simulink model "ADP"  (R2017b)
settings: Solver=FixedStepDiscrete  StartTime=0.0  StopTime=10.0  FixedStep=0.01  RelTol=1e-3  EnableMultiTasking=on
undefined symbols (not defined in the file): ADP050_RUNTIME_MS, ADP195_RUNTIME_MS, ADP_CONST100_NUMB, ADP_CONST2147483648_NUMB, ADP_CONST3_NUMB, ADP_CONST80_NUMB, ASWTYPE_FALSE, ASWTYPE_TRUE, CcADP_ABMDiagKL15DelayTi_ms, CcADP_ObcCmdto0Ti_ms, Enum_ADPStopChgReq, Enum_ISPDischgReq, Enum_LDPCC2St, Enum_MSMBMUState, Enum_ODPCCState, Enum_UDSPrjSel
libraries: AIWAYS_Powertrain_BMS_lib x68
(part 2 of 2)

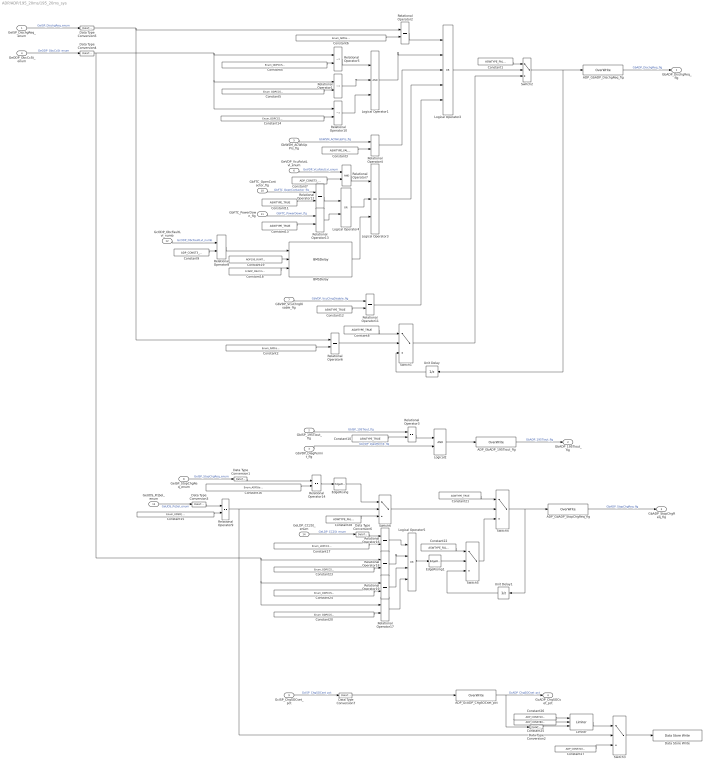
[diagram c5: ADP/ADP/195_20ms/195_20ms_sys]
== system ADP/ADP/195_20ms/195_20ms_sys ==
  GeISP_DischgReq_enum : Inport
  GbISP_195Tiout_flg : Inport  Port=2
  GbVDP_DiagPermit_flg : Inport  Port=3
  GeODP_ObcCcSt_enum : Inport  Port=4
  GbWSM_ACWkUpPrs_flg : Inport  Port=5
  GeVDP_VcuFalutLvl_enum : Inport  Port=6
  GbVDP_VcuChrgDisable_flg : Inport  Port=7
  GeISP_StopChgReq_enum : Inport  Port=8
  GcISP_ChgSOCset_pct : Inport  Port=9
  GbFTC_OpenContactor_flg : Inport  Port=10
  GbFTC_PowerDown_flg : Inport  Port=11
  GcODP_ObcFaultLvl_numb : Inport  Port=12
  GeUDS_PrjSel_enum : Inport  Port=13
  GeLDP_CC2St_enum : Inport  Port=14
  ADP_GbADP_195Tiout_flg : AIWAYS_Powertrain_BMS_lib/Signals/OverWrite  OverWrite_Value=CbADP_195TioutOvr_flg  OverWrite_flag=CbADP_195TioutOvrSwt_flg
  ADP_GbADP_DischgReq_flg : AIWAYS_Powertrain_BMS_lib/Signals/OverWrite  OverWrite_Value=CbADP_DischgReqOvr_flg  OverWrite_flag=CbADP_DischgReqOvrSwt_flg
  ADP_GbADP_StopChgReq_flg : AIWAYS_Powertrain_BMS_lib/Signals/OverWrite  OverWrite_Value=CbADP_StopChgReqOvr_flg  OverWrite_flag=CbADP_StopChgReqOvrSwt_flg
  ADP_GcADP_ChgSOCset_pct : AIWAYS_Powertrain_BMS_lib/Signals/OverWrite  OverWrite_Value=CcADP_ChgSOCsetOvr_pct  OverWrite_flag=CbADP_ChgSOCsetOvrSwt_flg
  BMSDelay : AIWAYS_Powertrain_BMS_lib/Debounce & Delay/BMSDelay
  Constant{1,3,22,28} (4 alike) : Constant  Value=ASWTYPE_FALSE
  Constant{8,10..13,21} (6 alike) : Constant  Value=ASWTYPE_TRUE
  Constant14 : Constant  Value=Enum_ODPCCState.Enum_ODPCCState_DisChrgConnect32A1000
  Constant15 : Constant  Value=Enum_UDSPrjSel.Enum_UDSPrjSel_891
  Constant16 : Constant  Value=Enum_ADPStopChgReq.Enum_ADPStopChgReq_StopChgReq
  Constant17 : Constant  Value=Enum_LDPCC2St.Enum_LDPCC2St_Connect
  Constant18 : Constant  Value=CcADP_ObcCmdto0Ti_ms
  Constant19 : Constant  Value=ADP195_RUNTIME_MS
  Constant2 : Constant  Value=Enum_ISPDischgReq.Enum_ISPDischgReq_V2XDischrg
  Constant20 : Constant  Value=Enum_ODPCCState.Enum_ODPCCState_ChrgConnect32A220
  Constant23 : Constant  Value=Enum_ODPCCState.Enum_ODPCCState_ChrgConnect10A1500
  Constant24 : Constant  Value=Enum_ODPCCState.Enum_ODPCCState_ChrgConnect16A680
  Constant25 : Constant  Value=ADP_CONST80_NUMB
  Constant26 : Constant  Value=ADP_CONST100_NUMB
  Constant27 : Constant  Value=ADP_CONST100_NUMB
  Constant4 : Constant  Value=Enum_ODPCCState.Enum_ODPCCState_DisChrgConnect10A2700
  Constant5 : Constant  Value=Enum_ODPCCState.Enum_ODPCCState_DisChrgConnect16A2000
  Constant6 : Constant  Value=Enum_ISPDischgReq.Enum_ISPDischgReq_QuitRequest
  Constant7 : Constant  Value=ADP_CONST3_NUMB
  Constant9 : Constant  Value=ADP_CONST3_NUMB
  Data Store Write : AIWAYS_Powertrain_BMS_lib/Signals/Data Store Write  DSW=EcNVM_ChrgPermitMaxSOC_pct
  Data Type Conversion{1..7} (7 alike) : DataTypeConversion
  EdgeRising : AIWAYS_Powertrain_BMS_lib/Logical Operators/EdgeRising
  EdgeRising1 : AIWAYS_Powertrain_BMS_lib/Logical Operators/EdgeRising
  Limiter : AIWAYS_Powertrain_BMS_lib/Nonlinear Blocks/Limiter
  Logical Operator1 : Logic  Inputs=3  AllPortsSameDT=off  OutDataTypeStr=boolean
  Logical Operator2 : Logic  Operator=OR  Inputs=5  AllPortsSameDT=off  OutDataTypeStr=boolean
  Logical Operator3 : Logic  Operator=OR  Inputs=3  AllPortsSameDT=off  OutDataTypeStr=boolean
  Logical Operator4 : Logic  Operator=OR  AllPortsSameDT=off  OutDataTypeStr=boolean
  Logical Operator5 : Logic  Operator=OR  Inputs=4  AllPortsSameDT=off  OutDataTypeStr=boolean
  Logical2 : Logic  OutDataTypeStr=boolean
  Relational Operator1 : RelationalOperator  Operator=~=  OutDataTypeStr=boolean
  Relational Operator10 : RelationalOperator  Operator=~=  OutDataTypeStr=boolean
  Relational Operator{2..4,6,8..9,11..14,16..19} (14 alike) : RelationalOperator  Operator===  OutDataTypeStr=boolean
  Relational Operator5 : RelationalOperator  Operator=~=  OutDataTypeStr=boolean
  Relational Operator7 : RelationalOperator  OutDataTypeStr=boolean
  Switch{1..6} (6 alike) : Switch  Criteria=u2 ~= 0
  Unit Delay : UnitDelay  SampleTime=-1  StateName=StateName
  Unit Delay1 : UnitDelay  SampleTime=-1  StateName=StateName
  GbADP_DischgReq_flg : Outport
  GbADP_195Tiout_flg : Outport  Port=2
  GbADP_StopChgReq_flg : Outport  Port=3
  GcADP_ChgSOCset_pct : Outport  Port=4
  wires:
  GbISP_195Tiout_flg/1 -> Relational Operator3/1  "GbISP_195Tiout_flg"
  GeISP_DischgReq_enum/1 -> Data Type Conversion5/1  "GeISP_DischgReq_enum"
  ADP_GbADP_DischgReq_flg/1 -> GbADP_DischgReq_flg/1  "GbADP_DischgReq_flg"
  GbVDP_DiagPermit_flg/1 -> Logical2/2  "GbVDP_DiagPermit_flg"
  Logical2/1 -> ADP_GbADP_195Tiout_flg/1
  Constant10/1 -> Relational Operator3/2
  Relational Operator3/1 -> Logical2/1
  ADP_GbADP_195Tiout_flg/1 -> GbADP_195Tiout_flg/1  "GbADP_195Tiout_flg"
  Relational Operator6/1 -> Switch1/2
  Constant2/1 -> Relational Operator6/2
  Constant8/1 -> Switch1/1
  Switch1/1 -> Switch2/3
  Constant1/1 -> Switch2/1
  Switch2/1 -> ADP_GbADP_DischgReq_flg/1, Unit Delay/1
  Unit Delay/1 -> Switch1/3
  Logical Operator2/1 -> Switch2/2
  Relational Operator5/1 -> Logical Operator1/1
  Constant4/1 -> Relational Operator5/2
  Constant14/1 -> Relational Operator10/2
  Relational Operator1/1 -> Logical Operator1/2
  Relational Operator10/1 -> Logical Operator1/3
  Constant5/1 -> Relational Operator1/2
  GeODP_ObcCcSt_enum/1 -> Data Type Conversion4/1  "GeODP_ObcCcSt_enum"
  Constant6/1 -> Relational Operator2/2
  GbWSM_ACWkUpPrs_flg/1 -> Relational Operator4/1  "GbWSM_ACWkUpPrs_flg"
  Constant3/1 -> Relational Operator4/2
  Relational Operator2/1 -> Logical Operator2/1
  Logical Operator1/1 -> Logical Operator2/2
  Relational Operator4/1 -> Logical Operator2/3
  GeVDP_VcuFalutLvl_enum/1 -> Relational Operator7/1  "GeVDP_VcuFalutLvl_enum"
  Constant7/1 -> Relational Operator7/2
  Relational Operator7/1 -> Logical Operator3/1
  Logical Operator4/1 -> Logical Operator3/2
  Logical Operator3/1 -> Logical Operator2/4
  GbVDP_VcuChrgDisable_flg/1 -> Relational Operator11/1  "GbVDP_VcuChrgDisable_flg"
  Constant12/1 -> Relational Operator11/2
  Relational Operator11/1 -> Logical Operator2/5
  Data Type Conversion5/1 -> Relational Operator6/1, Relational Operator2/1
  GeISP_StopChgReq_enum/1 -> Data Type Conversion1/1  "GeISP_StopChgReq_enum"
  GcISP_ChgSOCset_pct/1 -> Data Type Conversion7/1  "GcISP_ChgSOCset_pct"
  Data Type Conversion1/1 -> Relational Operator14/1
  ADP_GbADP_StopChgReq_flg/1 -> GbADP_StopChgReq_flg/1  "GbADP_StopChgReq_flg"
  Data Type Conversion7/1 -> ADP_GcADP_ChgSOCset_pct/1
  ADP_GcADP_ChgSOCset_pct/1 -> GcADP_ChgSOCset_pct/1, Data Type Conversion2/1  "GcADP_ChgSOCset_pct"
  GbFTC_OpenContactor_flg/1 -> Relational Operator12/1  "GbFTC_OpenContactor_flg"
  Relational Operator13/1 -> Logical Operator4/2
  Constant13/1 -> Relational Operator13/2
  Constant11/1 -> Relational Operator12/2
  GbFTC_PowerDown_flg/1 -> Relational Operator13/1  "GbFTC_PowerDown_flg"
  Relational Operator12/1 -> Logical Operator4/1
  GcODP_ObcFaultLvl_numb/1 -> Relational Operator8/1  "GcODP_ObcFaultLvl_numb"
  Relational Operator8/1 -> BMSDelay/1
  Constant9/1 -> Relational Operator8/2
  Constant19/1 -> BMSDelay/2
  Constant18/1 -> BMSDelay/3
  BMSDelay/1 -> Logical Operator3/3
  Data Type Conversion2/1 -> Limiter/3
  Constant15/1 -> Relational Operator9/2
  Data Type Conversion3/1 -> Relational Operator9/1
  GeUDS_PrjSel_enum/1 -> Data Type Conversion3/1  "GeUDS_PrjSel_enum"
  Relational Operator9/1 -> Switch3/2, Switch6/2
  Switch3/1 -> Data Store Write/1
  Constant27/1 -> Switch3/3
  Constant16/1 -> Relational Operator14/2
  Relational Operator14/1 -> EdgeRising/1
  Constant21/1 -> Switch4/1
  EdgeRising/1 -> Switch6/1
  Unit Delay1/1 -> Switch5/3
  Constant17/1 -> Relational Operator16/2
  EdgeRising1/1 -> Switch5/2
  Switch4/1 -> ADP_GbADP_StopChgReq_flg/1, Unit Delay1/1
  Relational Operator16/1 -> Logical Operator5/1
  Switch5/1 -> Switch4/3
  Constant22/1 -> Switch5/1
  Data Type Conversion6/1 -> Relational Operator16/1
  GeLDP_CC2St_enum/1 -> Data Type Conversion6/1  "GeLDP_CC2St_enum"
  Logical Operator5/1 -> EdgeRising1/1
  Relational Operator18/1 -> Logical Operator5/2
  Constant20/1 -> Relational Operator17/2
  Constant24/1 -> Relational Operator19/2
  Data Type Conversion4/1 -> Relational Operator18/1, Relational Operator17/1, Relational Operator19/1, Relational Operator5/1, Relational Operator10/1, Relational Operator1/1
  Constant23/1 -> Relational Operator18/2
  Relational Operator19/1 -> Logical Operator5/3
  Relational Operator17/1 -> Logical Operator5/4
  Limiter/1 -> Switch3/1
  Constant25/1 -> Limiter/2
  Constant26/1 -> Limiter/1
  Switch6/1 -> Switch4/2
  Constant28/1 -> Switch6/3

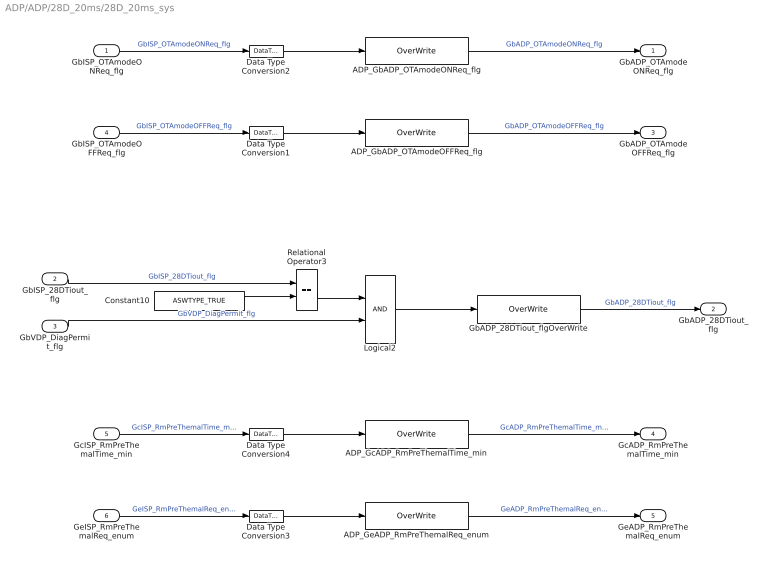
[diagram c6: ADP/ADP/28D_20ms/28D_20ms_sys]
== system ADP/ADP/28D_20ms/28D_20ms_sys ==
  GbISP_OTAmodeONReq_flg : Inport
  GbISP_28DTiout_flg : Inport  Port=2
  GbVDP_DiagPermit_flg : Inport  Port=3
  GbISP_OTAmodeOFFReq_flg : Inport  Port=4
  GcISP_RmPreThemalTime_min : Inport  Port=5
  GeISP_RmPreThemalReq_enum : Inport  Port=6
  ADP_GbADP_OTAmodeOFFReq_flg : AIWAYS_Powertrain_BMS_lib/Signals/OverWrite  OverWrite_Value=CbADP_OTAmodeOFFReqOvr_flg  OverWrite_flag=CbADP_OTAmodeOFFReqOvrSwt_flg
  ADP_GbADP_OTAmodeONReq_flg : AIWAYS_Powertrain_BMS_lib/Signals/OverWrite  OverWrite_Value=CbADP_OTAmodeONReqOvr_flg  OverWrite_flag=CbADP_OTAmodeONReqOvrSwt_flg
  ADP_GcADP_RmPreThemalTime_min : AIWAYS_Powertrain_BMS_lib/Signals/OverWrite  OverWrite_Value=CcADP_RmPreThemalTimeOvr_min  OverWrite_flag=CbADP_RmPreThemalTimeOvrSwt_flg
  ADP_GeADP_RmPreThemalReq_enum : AIWAYS_Powertrain_BMS_lib/Signals/OverWrite  OverWrite_Value=CeADP_RmPreThemalReqOvr_enum  OverWrite_flag=CbADP_RmPreThemalReqOvrSwt_flg
  Constant10 : Constant  Value=ASWTYPE_TRUE
  Data Type Conversion{1..4} (4 alike) : DataTypeConversion
  GbADP_28DTiout_flgOverWrite : AIWAYS_Powertrain_BMS_lib/Signals/OverWrite  OverWrite_Value=CbADP_28DTioutOvr_flg  OverWrite_flag=CbADP_28DTioutOvrSwt_flg
  Logical2 : Logic  OutDataTypeStr=boolean
  Relational Operator3 : RelationalOperator  Operator===  OutDataTypeStr=boolean
  GbADP_OTAmodeONReq_flg : Outport
  GbADP_28DTiout_flg : Outport  Port=2
  GbADP_OTAmodeOFFReq_flg : Outport  Port=3
  GcADP_RmPreThemalTime_min : Outport  Port=4
  GeADP_RmPreThemalReq_enum : Outport  Port=5
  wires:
  GbISP_OTAmodeONReq_flg/1 -> Data Type Conversion2/1  "GbISP_OTAmodeONReq_flg"
  GbISP_28DTiout_flg/1 -> Relational Operator3/1  "GbISP_28DTiout_flg"
  ADP_GbADP_OTAmodeONReq_flg/1 -> GbADP_OTAmodeONReq_flg/1  "GbADP_OTAmodeONReq_flg"
  GbVDP_DiagPermit_flg/1 -> Logical2/2  "GbVDP_DiagPermit_flg"
  Constant10/1 -> Relational Operator3/2
  Logical2/1 -> GbADP_28DTiout_flgOverWrite/1
  Relational Operator3/1 -> Logical2/1
  ADP_GbADP_OTAmodeOFFReq_flg/1 -> GbADP_OTAmodeOFFReq_flg/1  "GbADP_OTAmodeOFFReq_flg"
  GbISP_OTAmodeOFFReq_flg/1 -> Data Type Conversion1/1  "GbISP_OTAmodeOFFReq_flg"
  GbADP_28DTiout_flgOverWrite/1 -> GbADP_28DTiout_flg/1  "GbADP_28DTiout_flg"
  Data Type Conversion2/1 -> ADP_GbADP_OTAmodeONReq_flg/1
  Data Type Conversion1/1 -> ADP_GbADP_OTAmodeOFFReq_flg/1
  GeISP_RmPreThemalReq_enum/1 -> Data Type Conversion3/1  "GeISP_RmPreThemalReq_enum"
  Data Type Conversion4/1 -> ADP_GcADP_RmPreThemalTime_min/1
  Data Type Conversion3/1 -> ADP_GeADP_RmPreThemalReq_enum/1
  GcISP_RmPreThemalTime_min/1 -> Data Type Conversion4/1  "GcISP_RmPreThemalTime_min"
  ADP_GcADP_RmPreThemalTime_min/1 -> GcADP_RmPreThemalTime_min/1  "GcADP_RmPreThemalTime_min"
  ADP_GeADP_RmPreThemalReq_enum/1 -> GeADP_RmPreThemalReq_enum/1  "GeADP_RmPreThemalReq_enum"

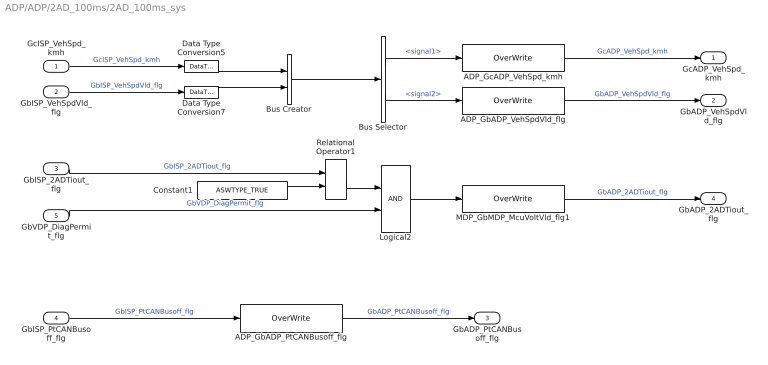
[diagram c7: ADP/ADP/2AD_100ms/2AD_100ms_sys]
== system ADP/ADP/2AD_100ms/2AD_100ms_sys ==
  GcISP_VehSpd_kmh : Inport
  GbISP_VehSpdVld_flg : Inport  Port=2
  GbISP_2ADTiout_flg : Inport  Port=3
  GbISP_PtCANBusoff_flg : Inport  Port=4
  GbVDP_DiagPermit_flg : Inport  Port=5
  ADP_GbADP_PtCANBusoff_flg : AIWAYS_Powertrain_BMS_lib/Signals/OverWrite  OverWrite_Value=CbADP_PtCANBusoffOvr_flg  OverWrite_flag=CbADP_PtCANBusoffOvrSwt_flg
  ADP_GbADP_VehSpdVld_flg : AIWAYS_Powertrain_BMS_lib/Signals/OverWrite  OverWrite_Value=CbADP_VehSpdVldOvr_flg  OverWrite_flag=CbADP_VehSpdVldOvrSwt_flg
  ADP_GcADP_VehSpd_kmh : AIWAYS_Powertrain_BMS_lib/Signals/OverWrite  OverWrite_Value=CcADP_VehSpdOvr_kmh  OverWrite_flag=CbADP_VehSpdOvrSwt_flg
  Bus Creator : BusCreator  Inputs=2
  Bus Selector : BusSelector  OutputSignals=signal1,signal2
  Constant1 : Constant  Value=ASWTYPE_TRUE
  Data Type Conversion5 : DataTypeConversion
  Data Type Conversion7 : DataTypeConversion
  Logical2 : Logic  OutDataTypeStr=boolean
  MDP_GbMDP_McuVoltVld_flg1 : AIWAYS_Powertrain_BMS_lib/Signals/OverWrite  OverWrite_Value=CbADP_2ADTioutOvr_flg  OverWrite_flag=CbADP_2ADTioutOvrSwt_flg
  Relational Operator1 : RelationalOperator  Operator===  OutDataTypeStr=boolean
  GcADP_VehSpd_kmh : Outport
  GbADP_VehSpdVld_flg : Outport  Port=2
  GbADP_PtCANBusoff_flg : Outport  Port=3
  GbADP_2ADTiout_flg : Outport  Port=4
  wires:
  Bus Selector/2 -> ADP_GbADP_VehSpdVld_flg/1  "<signal2>"
  Data Type Conversion5/1 -> Bus Creator/1
  Data Type Conversion7/1 -> Bus Creator/2
  Bus Creator/1 -> Bus Selector/1
  Bus Selector/1 -> ADP_GcADP_VehSpd_kmh/1  "<signal1>"
  GcISP_VehSpd_kmh/1 -> Data Type Conversion5/1  "GcISP_VehSpd_kmh"
  GbISP_VehSpdVld_flg/1 -> Data Type Conversion7/1  "GbISP_VehSpdVld_flg"
  GbISP_2ADTiout_flg/1 -> Relational Operator1/1  "GbISP_2ADTiout_flg"
  ADP_GcADP_VehSpd_kmh/1 -> GcADP_VehSpd_kmh/1  "GcADP_VehSpd_kmh"
  ADP_GbADP_VehSpdVld_flg/1 -> GbADP_VehSpdVld_flg/1  "GbADP_VehSpdVld_flg"
  ADP_GbADP_PtCANBusoff_flg/1 -> GbADP_PtCANBusoff_flg/1  "GbADP_PtCANBusoff_flg"
  GbISP_PtCANBusoff_flg/1 -> ADP_GbADP_PtCANBusoff_flg/1  "GbISP_PtCANBusoff_flg"
  Logical2/1 -> MDP_GbMDP_McuVoltVld_flg1/1
  GbVDP_DiagPermit_flg/1 -> Logical2/2  "GbVDP_DiagPermit_flg"
  MDP_GbMDP_McuVoltVld_flg1/1 -> GbADP_2ADTiout_flg/1  "GbADP_2ADTiout_flg"
  Constant1/1 -> Relational Operator1/2
  Relational Operator1/1 -> Logical2/1

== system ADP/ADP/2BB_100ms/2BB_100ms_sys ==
  GcISP_EnvT_C : Inport
  GbISP_2BBTiout_flg : Inport  Port=2
  GbVDP_DiagPermit_flg : Inport  Port=3
  ADP_GbADP_2BBTiout_flg : AIWAYS_Powertrain_BMS_lib/Signals/OverWrite  OverWrite_Value=CbADP_2BBTioutOvr_flg  OverWrite_flag=CbADP_2BBTioutOvrSwt_flg
  ADP_GcADP_EnvT_C : AIWAYS_Powertrain_BMS_lib/Signals/OverWrite  OverWrite_Value=CcADP_EnvTOvr_C  OverWrite_flag=CbADP_EnvTOvrSwt_flg
  Constant1 : Constant  Value=ASWTYPE_TRUE
  Data Type Conversion5 : DataTypeConversion
  Logical2 : Logic  OutDataTypeStr=boolean
  Relational Operator1 : RelationalOperator  Operator===  OutDataTypeStr=boolean
  GcADP_EnvT_C : Outport
  GbADP_2BBTiout_flg : Outport  Port=2
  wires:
  GbISP_2BBTiout_flg/1 -> Relational Operator1/1  "GbISP_2BBTiout_flg"
  GcISP_EnvT_C/1 -> Data Type Conversion5/1  "GcISP_EnvT_C"
  Data Type Conversion5/1 -> ADP_GcADP_EnvT_C/1
  ADP_GcADP_EnvT_C/1 -> GcADP_EnvT_C/1  "GcADP_EnvT_C"
  Logical2/1 -> ADP_GbADP_2BBTiout_flg/1
  GbVDP_DiagPermit_flg/1 -> Logical2/2  "GbVDP_DiagPermit_flg"
  Constant1/1 -> Relational Operator1/2
  Relational Operator1/1 -> Logical2/1
  ADP_GbADP_2BBTiout_flg/1 -> GbADP_2BBTiout_flg/1  "GbADP_2BBTiout_flg"

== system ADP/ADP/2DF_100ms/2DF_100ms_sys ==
  GcISP_AcmDist_numb : Inport
  GbISP_AcmDistVld_flg : Inport  Port=2
  GbISP_2DFTiout_flg : Inport  Port=3
  GbVDP_DiagPermit_flg : Inport  Port=4
  ADP_GbADP_2DFTiout_flg : AIWAYS_Powertrain_BMS_lib/Signals/OverWrite  OverWrite_Value=CbADP_2DFTioutOvr_flg  OverWrite_flag=CbADP_2DFTioutOvrSwt_flg
  ADP_GbADP_AcmDistVld_flg : AIWAYS_Powertrain_BMS_lib/Signals/OverWrite  OverWrite_Value=CbADP_AcmDistVldOvr_flg  OverWrite_flag=CbADP_AcmDistVldOvrSwt_flg
  ADP_GcADP_AcmDist_numb : AIWAYS_Powertrain_BMS_lib/Signals/OverWrite  OverWrite_Value=CcADP_AcmDistOvr_numb  OverWrite_flag=CbADP_AcmDistOvrSwt_flg
  Bus Creator : BusCreator  Inputs=2
  Bus Selector : BusSelector  OutputSignals=signal1,signal2
  Constant3 : Constant  Value=ASWTYPE_TRUE
  Data Type Conversion5 : DataTypeConversion
  Data Type Conversion7 : DataTypeConversion
  Logical2 : Logic  OutDataTypeStr=boolean
  Relational Operator1 : RelationalOperator  Operator===  OutDataTypeStr=boolean
  GcADP_AcmDist_numb : Outport
  GbADP_AcmDistVld_flg : Outport  Port=2
  GbADP_2DFTiout_flg : Outport  Port=3
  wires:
  Bus Selector/1 -> ADP_GcADP_AcmDist_numb/1  "<signal1>"
  Bus Selector/2 -> ADP_GbADP_AcmDistVld_flg/1  "<signal2>"
  Bus Creator/1 -> Bus Selector/1
  Data Type Conversion7/1 -> Bus Creator/2
  Data Type Conversion5/1 -> Bus Creator/1
  GcISP_AcmDist_numb/1 -> Data Type Conversion5/1  "GcISP_AcmDist_numb"
  GbISP_AcmDistVld_flg/1 -> Data Type Conversion7/1  "GbISP_AcmDistVld_flg"
  GbISP_2DFTiout_flg/1 -> Relational Operator1/1  "GbISP_2DFTiout_flg"
  ADP_GcADP_AcmDist_numb/1 -> GcADP_AcmDist_numb/1  "GcADP_AcmDist_numb"
  ADP_GbADP_AcmDistVld_flg/1 -> GbADP_AcmDistVld_flg/1  "GbADP_AcmDistVld_flg"
  GbVDP_DiagPermit_flg/1 -> Logical2/2  "GbVDP_DiagPermit_flg"
  Logical2/1 -> ADP_GbADP_2DFTiout_flg/1
  Constant3/1 -> Relational Operator1/2
  Relational Operator1/1 -> Logical2/1
  ADP_GbADP_2DFTiout_flg/1 -> GbADP_2DFTiout_flg/1  "GbADP_2DFTiout_flg"

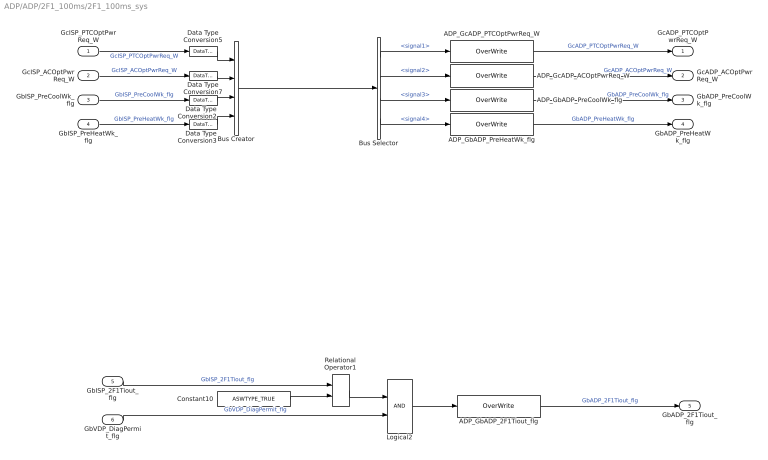
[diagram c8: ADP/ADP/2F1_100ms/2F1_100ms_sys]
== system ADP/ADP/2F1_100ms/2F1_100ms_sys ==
  GcISP_PTCOptPwrReq_W : Inport
  GcISP_ACOptPwrReq_W : Inport  Port=2
  GbISP_PreCoolWk_flg : Inport  Port=3
  GbISP_PreHeatWk_flg : Inport  Port=4
  GbISP_2F1Tiout_flg : Inport  Port=5
  GbVDP_DiagPermit_flg : Inport  Port=6
  ADP_GbADP_2F1Tiout_flg : AIWAYS_Powertrain_BMS_lib/Signals/OverWrite  OverWrite_Value=CbADP_2F1TioutOvr_flg  OverWrite_flag=CbADP_2F1TioutOvrSwt_flg
  ADP_GbADP_PreCoolWk_flg : AIWAYS_Powertrain_BMS_lib/Signals/OverWrite  OverWrite_Value=CbADP_PreCoolWkOvr_flg  OverWrite_flag=CbADP_PreCoolWkOvrSwt_flg
  ADP_GbADP_PreHeatWk_flg : AIWAYS_Powertrain_BMS_lib/Signals/OverWrite  OverWrite_Value=CbADP_PreHeatWkOvr_flg  OverWrite_flag=CbADP_PreHeatWkOvrSwt_flg
  ADP_GcADP_ACOptPwrReq_W : AIWAYS_Powertrain_BMS_lib/Signals/OverWrite  OverWrite_Value=CcADP_ACOptPwrReqOvr_W  OverWrite_flag=CbADP_ACOptPwrReqOvrSwt_flg
  ADP_GcADP_PTCOptPwrReq_W : AIWAYS_Powertrain_BMS_lib/Signals/OverWrite  OverWrite_Value=CcADP_PTCOptPwrReqOvr_W  OverWrite_flag=CbADP_PTCOptPwrReqOvrSwt_flg
  Bus Creator : BusCreator  Inputs=4
  Bus Selector : BusSelector  OutputSignals=signal1,signal2,signal3,signal4
  Constant10 : Constant  Value=ASWTYPE_TRUE
  Data Type Conversion{2..3,5,7} (4 alike) : DataTypeConversion
  Logical2 : Logic  OutDataTypeStr=boolean
  Relational Operator1 : RelationalOperator  Operator===  OutDataTypeStr=boolean
  GcADP_PTCOptPwrReq_W : Outport
  GcADP_ACOptPwrReq_W : Outport  Port=2
  GbADP_PreCoolWk_flg : Outport  Port=3
  GbADP_PreHeatWk_flg : Outport  Port=4
  GbADP_2F1Tiout_flg : Outport  Port=5
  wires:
  Bus Creator/1 -> Bus Selector/1
  Data Type Conversion7/1 -> Bus Creator/2
  Data Type Conversion5/1 -> Bus Creator/1
  GcISP_ACOptPwrReq_W/1 -> Data Type Conversion7/1  "GcISP_ACOptPwrReq_W"
  GcISP_PTCOptPwrReq_W/1 -> Data Type Conversion5/1  "GcISP_PTCOptPwrReq_W"
  GbISP_PreCoolWk_flg/1 -> Data Type Conversion2/1  "GbISP_PreCoolWk_flg"
  GbISP_PreHeatWk_flg/1 -> Data Type Conversion3/1  "GbISP_PreHeatWk_flg"
  GbISP_2F1Tiout_flg/1 -> Relational Operator1/1  "GbISP_2F1Tiout_flg"
  ADP_GcADP_PTCOptPwrReq_W/1 -> GcADP_PTCOptPwrReq_W/1  "GcADP_PTCOptPwrReq_W"
  ADP_GcADP_ACOptPwrReq_W/1 -> GcADP_ACOptPwrReq_W/1  "GcADP_ACOptPwrReq_W"
  ADP_GbADP_PreCoolWk_flg/1 -> GbADP_PreCoolWk_flg/1  "GbADP_PreCoolWk_flg"
  ADP_GbADP_PreHeatWk_flg/1 -> GbADP_PreHeatWk_flg/1  "GbADP_PreHeatWk_flg"
  Bus Selector/1 -> ADP_GcADP_PTCOptPwrReq_W/1  "<signal1>"
  Bus Selector/2 -> ADP_GcADP_ACOptPwrReq_W/1  "<signal2>"
  Bus Selector/3 -> ADP_GbADP_PreCoolWk_flg/1  "<signal3>"
  Bus Selector/4 -> ADP_GbADP_PreHeatWk_flg/1  "<signal4>"
  Data Type Conversion2/1 -> Bus Creator/3
  Data Type Conversion3/1 -> Bus Creator/4
  Logical2/1 -> ADP_GbADP_2F1Tiout_flg/1
  GbVDP_DiagPermit_flg/1 -> Logical2/2  "GbVDP_DiagPermit_flg"
  Relational Operator1/1 -> Logical2/1
  Constant10/1 -> Relational Operator1/2
  ADP_GbADP_2F1Tiout_flg/1 -> GbADP_2F1Tiout_flg/1  "GbADP_2F1Tiout_flg"

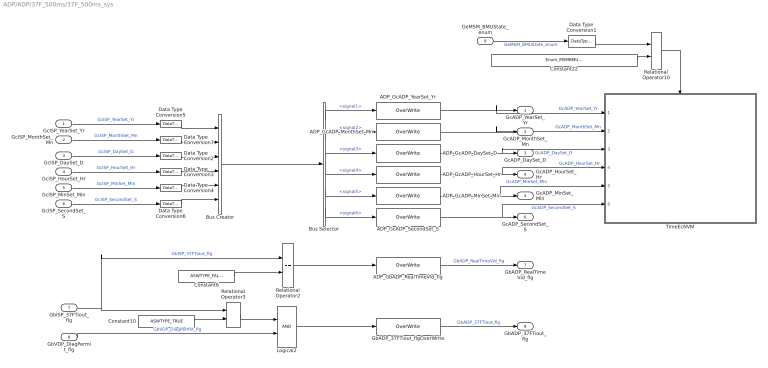
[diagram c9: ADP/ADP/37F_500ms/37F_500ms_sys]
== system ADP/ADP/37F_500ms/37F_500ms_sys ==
  GcISP_YearSet_Yr : Inport
  GcISP_MonthSet_Mn : Inport  Port=2
  GcISP_DaySet_D : Inport  Port=3
  GcISP_HourSet_Hr : Inport  Port=4
  GcISP_MinSet_Min : Inport  Port=5
  GcISP_SecondSet_S : Inport  Port=6
  GbISP_37FTiout_flg : Inport  Port=7
  GbVDP_DiagPermit_flg : Inport  Port=8
  GeMSM_BMUState_enum : Inport  Port=9
  ADP_GbADP_RealTimeVld_flg : AIWAYS_Powertrain_BMS_lib/Signals/OverWrite  OverWrite_Value=CbADP_RealTimeVldOvr_flg  OverWrite_flag=CbADP_RealTimeVldOvrSwt_flg
  ADP_GcADP_DaySet_D : AIWAYS_Powertrain_BMS_lib/Signals/OverWrite  OverWrite_Value=CcADP_DaySetOvr_D  OverWrite_flag=CbADP_DaySetOvrSwt_flg
  ADP_GcADP_HourSet_Hr : AIWAYS_Powertrain_BMS_lib/Signals/OverWrite  OverWrite_Value=CcADP_HourSetOvr_Hr  OverWrite_flag=CbADP_HourSetOvrSwt_flg
  ADP_GcADP_MinSet_Min : AIWAYS_Powertrain_BMS_lib/Signals/OverWrite  OverWrite_Value=CcADP_MinSetOvr_Min  OverWrite_flag=CbADP_MinSetOvrSwt_flg
  ADP_GcADP_MonthSet_Mn : AIWAYS_Powertrain_BMS_lib/Signals/OverWrite  OverWrite_Value=CcADP_MonthSetOvr_Mn  OverWrite_flag=CbADP_MonthSetOvrSwt_flg
  ADP_GcADP_SecondSet_S : AIWAYS_Powertrain_BMS_lib/Signals/OverWrite  OverWrite_Value=CcADP_SecondSetOvr_S  OverWrite_flag=CbADP_SecondSetOvrSwt_flg
  ADP_GcADP_YearSet_Yr : AIWAYS_Powertrain_BMS_lib/Signals/OverWrite  OverWrite_Value=CcADP_YearSetOvr_Yr  OverWrite_flag=CbADP_YearSetOvrSwt_flg
  Bus Creator : BusCreator  Inputs=6
  Bus Selector : BusSelector  OutputSignals=signal1,signal2,signal3,signal4,signal5,signal6
  Constant10 : Constant  Value=ASWTYPE_TRUE
  Constant22 : Constant  Value=Enum_MSMBMUState.Enum_MSMBMUState_Shutdown
  Constant6 : Constant  Value=ASWTYPE_FALSE
  Data Type Conversion{1..7} (7 alike) : DataTypeConversion
  GbADP_37FTiout_flgOverWrite : AIWAYS_Powertrain_BMS_lib/Signals/OverWrite  OverWrite_Value=CbADP_37FTioutOvr_flg  OverWrite_flag=CbADP_37FTioutOvrSwt_flg
  Logical2 : Logic  OutDataTypeStr=boolean
  Relational Operator10 : RelationalOperator  Operator===  OutDataTypeStr=boolean
  Relational Operator2 : RelationalOperator  Operator===  OutDataTypeStr=boolean
  Relational Operator3 : RelationalOperator  Operator===  OutDataTypeStr=boolean
  TimeEcNVM : Subsystem
  GcADP_YearSet_Yr : Outport
  GcADP_MonthSet_Mn : Outport  Port=2
  GcADP_DaySet_D : Outport  Port=3
  GcADP_HourSet_Hr : Outport  Port=4
  GcADP_MinSet_Min : Outport  Port=5
  GcADP_SecondSet_S : Outport  Port=6
  GbADP_RealTimeVld_flg : Outport  Port=7
  GbADP_37FTiout_flg : Outport  Port=8
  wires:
  Data Type Conversion7/1 -> Bus Creator/2
  Data Type Conversion5/1 -> Bus Creator/1
  Data Type Conversion2/1 -> Bus Creator/3
  Data Type Conversion3/1 -> Bus Creator/4
  Data Type Conversion6/1 -> Bus Creator/6
  Data Type Conversion4/1 -> Bus Creator/5
  Bus Creator/1 -> Bus Selector/1
  Bus Selector/1 -> ADP_GcADP_YearSet_Yr/1  "<signal1>"
  ADP_GcADP_YearSet_Yr/1 -> TimeEcNVM/1(GcADP_YearSet_Yr), GcADP_YearSet_Yr/1  "GcADP_YearSet_Yr"
  ADP_GcADP_MonthSet_Mn/1 -> TimeEcNVM/2(GcADP_MonthSet_Mn), GcADP_MonthSet_Mn/1  "GcADP_MonthSet_Mn"
  Bus Selector/2 -> ADP_GcADP_MonthSet_Mn/1  "<signal2>"
  Bus Selector/3 -> ADP_GcADP_DaySet_D/1  "<signal3>"
  ADP_GcADP_DaySet_D/1 -> TimeEcNVM/3(GcADP_DaySet_D), GcADP_DaySet_D/1  "GcADP_DaySet_D"
  ADP_GcADP_HourSet_Hr/1 -> TimeEcNVM/4(GcADP_HourSet_Hr), GcADP_HourSet_Hr/1  "GcADP_HourSet_Hr"
  ADP_GcADP_MinSet_Min/1 -> TimeEcNVM/5(GcADP_MinSet_Min), GcADP_MinSet_Min/1  "GcADP_MinSet_Min"
  ADP_GcADP_SecondSet_S/1 -> TimeEcNVM/6(GcADP_SecondSet_S), GcADP_SecondSet_S/1  "GcADP_SecondSet_S"
  Bus Selector/4 -> ADP_GcADP_HourSet_Hr/1  "<signal4>"
  Bus Selector/5 -> ADP_GcADP_MinSet_Min/1  "<signal5>"
  Bus Selector/6 -> ADP_GcADP_SecondSet_S/1  "<signal6>"
  ADP_GbADP_RealTimeVld_flg/1 -> GbADP_RealTimeVld_flg/1  "GbADP_RealTimeVld_flg"
  GcISP_YearSet_Yr/1 -> Data Type Conversion5/1  "GcISP_YearSet_Yr"
  GcISP_MonthSet_Mn/1 -> Data Type Conversion7/1  "GcISP_MonthSet_Mn"
  GcISP_DaySet_D/1 -> Data Type Conversion2/1  "GcISP_DaySet_D"
  GcISP_HourSet_Hr/1 -> Data Type Conversion3/1  "GcISP_HourSet_Hr"
  GcISP_MinSet_Min/1 -> Data Type Conversion4/1  "GcISP_MinSet_Min"
  GcISP_SecondSet_S/1 -> Data Type Conversion6/1  "GcISP_SecondSet_S"
  GbVDP_DiagPermit_flg/1 -> Logical2/2  "GbVDP_DiagPermit_flg"
  Logical2/1 -> GbADP_37FTiout_flgOverWrite/1
  Constant10/1 -> Relational Operator3/2
  Relational Operator3/1 -> Logical2/1
  GbADP_37FTiout_flgOverWrite/1 -> GbADP_37FTiout_flg/1  "GbADP_37FTiout_flg"
  Relational Operator2/1 -> ADP_GbADP_RealTimeVld_flg/1
  Constant6/1 -> Relational Operator2/2
  GbISP_37FTiout_flg/1 -> Relational Operator2/1, Relational Operator3/1  "GbISP_37FTiout_flg"
  GeMSM_BMUState_enum/1 -> Data Type Conversion1/1  "GeMSM_BMUState_enum"
  Relational Operator10/1 -> TimeEcNVM/Enable
  Data Type Conversion1/1 -> Relational Operator10/1
  Constant22/1 -> Relational Operator10/2

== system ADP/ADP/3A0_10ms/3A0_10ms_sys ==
  GcISP_CsDataVer_numb : Inport
  GcISP_CsDataCrc_numb : Inport  Port=2
  ADP_GcADP_CsDataCrc_numb : AIWAYS_Powertrain_BMS_lib/Signals/OverWrite  OverWrite_Value=CcADP_CsDataCrcOvr_numb  OverWrite_flag=CbADP_CsDataCrcOvrSwt_flg
  ADP_GcADP_CsDataVer_numb : AIWAYS_Powertrain_BMS_lib/Signals/OverWrite  OverWrite_Value=CcADP_CsDataVerOvr_numb  OverWrite_flag=CbADP_CsDataVerOvrSwt_flg
  Data Type Conversion1 : DataTypeConversion
  Data Type Conversion2 : DataTypeConversion
  GcADP_CsDataVer_numb : Outport
  GcADP_CsDataCrc_numb : Outport  Port=2
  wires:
  GcISP_CsDataVer_numb/1 -> Data Type Conversion2/1  "GcISP_CsDataVer_numb"
  GcISP_CsDataCrc_numb/1 -> Data Type Conversion1/1  "GcISP_CsDataCrc_numb"
  Data Type Conversion2/1 -> ADP_GcADP_CsDataVer_numb/1
  Data Type Conversion1/1 -> ADP_GcADP_CsDataCrc_numb/1
  ADP_GcADP_CsDataVer_numb/1 -> GcADP_CsDataVer_numb/1  "GcADP_CsDataVer_numb"
  ADP_GcADP_CsDataCrc_numb/1 -> GcADP_CsDataCrc_numb/1  "GcADP_CsDataCrc_numb"

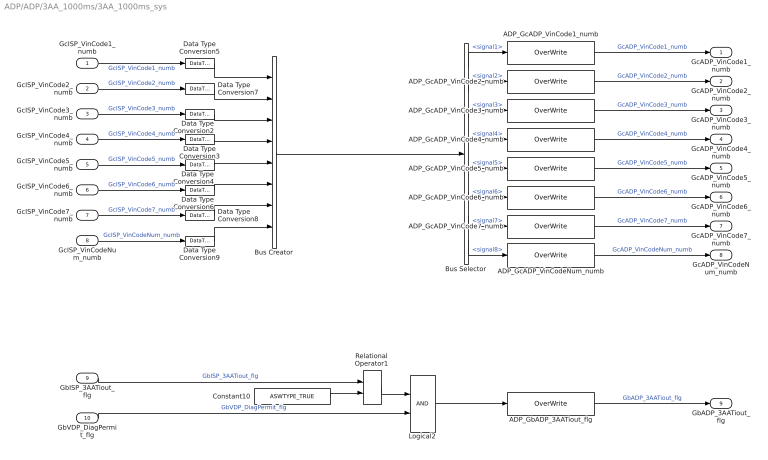
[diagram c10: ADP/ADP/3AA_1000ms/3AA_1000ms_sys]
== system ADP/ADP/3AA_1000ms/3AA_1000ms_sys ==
  GcISP_VinCode1_numb : Inport
  GcISP_VinCode2_numb : Inport  Port=2
  GcISP_VinCode3_numb : Inport  Port=3
  GcISP_VinCode4_numb : Inport  Port=4
  GcISP_VinCode5_numb : Inport  Port=5
  GcISP_VinCode6_numb : Inport  Port=6
  GcISP_VinCode7_numb : Inport  Port=7
  GcISP_VinCodeNum_numb : Inport  Port=8
  GbISP_3AATiout_flg : Inport  Port=9
  GbVDP_DiagPermit_flg : Inport  Port=10
  ADP_GbADP_3AATiout_flg : AIWAYS_Powertrain_BMS_lib/Signals/OverWrite  OverWrite_Value=CbADP_3AATioutOvr_flg  OverWrite_flag=CbADP_3AATioutOvrSwt_flg
  ADP_GcADP_VinCode1_numb : AIWAYS_Powertrain_BMS_lib/Signals/OverWrite  OverWrite_Value=CcADP_VinCode1Ovr_numb  OverWrite_flag=CbADP_VinCode1OvrSwt_flg
  ADP_GcADP_VinCode2_numb : AIWAYS_Powertrain_BMS_lib/Signals/OverWrite  OverWrite_Value=CcADP_VinCode2Ovr_numb  OverWrite_flag=CbADP_VinCode2OvrSwt_flg
  ADP_GcADP_VinCode3_numb : AIWAYS_Powertrain_BMS_lib/Signals/OverWrite  OverWrite_Value=CcADP_VinCode3Ovr_numb  OverWrite_flag=CbADP_VinCode3OvrSwt_flg
  ADP_GcADP_VinCode4_numb : AIWAYS_Powertrain_BMS_lib/Signals/OverWrite  OverWrite_Value=CcADP_VinCode4Ovr_numb  OverWrite_flag=CbADP_VinCode4OvrSwt_flg
  ADP_GcADP_VinCode5_numb : AIWAYS_Powertrain_BMS_lib/Signals/OverWrite  OverWrite_Value=CcADP_VinCode5Ovr_numb  OverWrite_flag=CbADP_VinCode5OvrSwt_flg
  ADP_GcADP_VinCode6_numb : AIWAYS_Powertrain_BMS_lib/Signals/OverWrite  OverWrite_Value=CcADP_VinCode6Ovr_numb  OverWrite_flag=CbADP_VinCode6OvrSwt_flg
  ADP_GcADP_VinCode7_numb : AIWAYS_Powertrain_BMS_lib/Signals/OverWrite  OverWrite_Value=CcADP_VinCode7Ovr_numb  OverWrite_flag=CbADP_VinCode7OvrSwt_flg
  ADP_GcADP_VinCodeNum_numb : AIWAYS_Powertrain_BMS_lib/Signals/OverWrite  OverWrite_Value=CcADP_VinCodeNumOvr_numb  OverWrite_flag=CbADP_VinCodeNumOvrSwt_flg
  Bus Creator : BusCreator  Inputs=8
  Bus Selector : BusSelector  OutputSignals=signal1,signal2,signal3,signal4,signal5,signal6,signal7,signal8
  Constant10 : Constant  Value=ASWTYPE_TRUE
  Data Type Conversion{2..9} (8 alike) : DataTypeConversion
  Logical2 : Logic  OutDataTypeStr=boolean
  Relational Operator1 : RelationalOperator  Operator===  OutDataTypeStr=boolean
  GcADP_VinCode1_numb : Outport
  GcADP_VinCode2_numb : Outport  Port=2
  GcADP_VinCode3_numb : Outport  Port=3
  GcADP_VinCode4_numb : Outport  Port=4
  GcADP_VinCode5_numb : Outport  Port=5
  GcADP_VinCode6_numb : Outport  Port=6
  GcADP_VinCode7_numb : Outport  Port=7
  GcADP_VinCodeNum_numb : Outport  Port=8
  GbADP_3AATiout_flg : Outport  Port=9
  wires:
  Data Type Conversion7/1 -> Bus Creator/2
  Data Type Conversion5/1 -> Bus Creator/1
  GcISP_VinCode1_numb/1 -> Data Type Conversion5/1  "GcISP_VinCode1_numb"
  GcISP_VinCode2_numb/1 -> Data Type Conversion7/1  "GcISP_VinCode2_numb"
  Data Type Conversion2/1 -> Bus Creator/3
  Data Type Conversion3/1 -> Bus Creator/4
  Data Type Conversion4/1 -> Bus Creator/5
  Data Type Conversion6/1 -> Bus Creator/6
  Data Type Conversion8/1 -> Bus Creator/7
  Data Type Conversion9/1 -> Bus Creator/8
  GcISP_VinCode5_numb/1 -> Data Type Conversion4/1  "GcISP_VinCode5_numb"
  GcISP_VinCode4_numb/1 -> Data Type Conversion3/1  "GcISP_VinCode4_numb"
  GcISP_VinCode3_numb/1 -> Data Type Conversion2/1  "GcISP_VinCode3_numb"
  GcISP_VinCode6_numb/1 -> Data Type Conversion6/1  "GcISP_VinCode6_numb"
  GcISP_VinCode7_numb/1 -> Data Type Conversion8/1  "GcISP_VinCode7_numb"
  GcISP_VinCodeNum_numb/1 -> Data Type Conversion9/1  "GcISP_VinCodeNum_numb"
  Bus Creator/1 -> Bus Selector/1
  GbISP_3AATiout_flg/1 -> Relational Operator1/1  "GbISP_3AATiout_flg"
  ADP_GcADP_VinCodeNum_numb/1 -> GcADP_VinCodeNum_numb/1  "GcADP_VinCodeNum_numb"
  ADP_GcADP_VinCode7_numb/1 -> GcADP_VinCode7_numb/1  "GcADP_VinCode7_numb"
  ADP_GcADP_VinCode6_numb/1 -> GcADP_VinCode6_numb/1  "GcADP_VinCode6_numb"
  ADP_GcADP_VinCode5_numb/1 -> GcADP_VinCode5_numb/1  "GcADP_VinCode5_numb"
  ADP_GcADP_VinCode4_numb/1 -> GcADP_VinCode4_numb/1  "GcADP_VinCode4_numb"
  ADP_GcADP_VinCode3_numb/1 -> GcADP_VinCode3_numb/1  "GcADP_VinCode3_numb"
  ADP_GcADP_VinCode2_numb/1 -> GcADP_VinCode2_numb/1  "GcADP_VinCode2_numb"
  ADP_GcADP_VinCode1_numb/1 -> GcADP_VinCode1_numb/1  "GcADP_VinCode1_numb"
  Bus Selector/1 -> ADP_GcADP_VinCode1_numb/1  "<signal1>"
  Bus Selector/2 -> ADP_GcADP_VinCode2_numb/1  "<signal2>"
  Bus Selector/3 -> ADP_GcADP_VinCode3_numb/1  "<signal3>"
  Bus Selector/4 -> ADP_GcADP_VinCode4_numb/1  "<signal4>"
  Bus Selector/5 -> ADP_GcADP_VinCode5_numb/1  "<signal5>"
  Bus Selector/6 -> ADP_GcADP_VinCode6_numb/1  "<signal6>"
  Bus Selector/7 -> ADP_GcADP_VinCode7_numb/1  "<signal7>"
  Bus Selector/8 -> ADP_GcADP_VinCodeNum_numb/1  "<signal8>"
  Constant10/1 -> Relational Operator1/2
  GbVDP_DiagPermit_flg/1 -> Logical2/2  "GbVDP_DiagPermit_flg"
  Logical2/1 -> ADP_GbADP_3AATiout_flg/1
  Relational Operator1/1 -> Logical2/1
  ADP_GbADP_3AATiout_flg/1 -> GbADP_3AATiout_flg/1  "GbADP_3AATiout_flg"

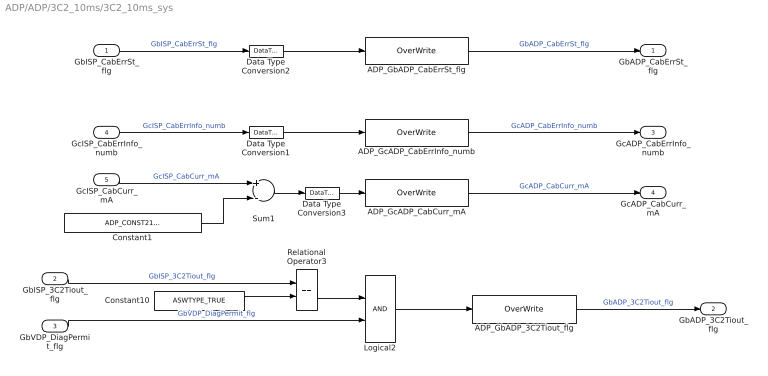
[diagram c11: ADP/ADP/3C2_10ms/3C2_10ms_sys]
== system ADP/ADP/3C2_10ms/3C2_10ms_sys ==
  GbISP_CabErrSt_flg : Inport
  GbISP_3C2Tiout_flg : Inport  Port=2
  GbVDP_DiagPermit_flg : Inport  Port=3
  GcISP_CabErrInfo_numb : Inport  Port=4
  GcISP_CabCurr_mA : Inport  Port=5
  ADP_GbADP_3C2Tiout_flg : AIWAYS_Powertrain_BMS_lib/Signals/OverWrite  OverWrite_Value=CbADP_3C2TioutOvr_flg  OverWrite_flag=CbADP_3C2TioutOvrSwt_flg
  ADP_GbADP_CabErrSt_flg : AIWAYS_Powertrain_BMS_lib/Signals/OverWrite  OverWrite_Value=CbADP_CabErrStOvr_flg  OverWrite_flag=CbADP_CabErrStOvrSwt_flg
  ADP_GcADP_CabCurr_mA : AIWAYS_Powertrain_BMS_lib/Signals/OverWrite  OverWrite_Value=CcADP_CabCurrOvr_mA  OverWrite_flag=CbADP_CabCurrOvrSwt_flg
  ADP_GcADP_CabErrInfo_numb : AIWAYS_Powertrain_BMS_lib/Signals/OverWrite  OverWrite_Value=CcADP_CabErrInfoOvr_numb  OverWrite_flag=CbADP_CabErrInfoOvrSwt_flg
  Constant1 : Constant  Value=ADP_CONST2147483648_NUMB
  Constant10 : Constant  Value=ASWTYPE_TRUE
  Data Type Conversion1 : DataTypeConversion
  Data Type Conversion2 : DataTypeConversion
  Data Type Conversion3 : DataTypeConversion
  Logical2 : Logic  OutDataTypeStr=boolean
  Relational Operator3 : RelationalOperator  Operator===  OutDataTypeStr=boolean
  Sum1 : Sum  Inputs=+-  OutDataTypeStr=int32  RndMeth=Zero
  GbADP_CabErrSt_flg : Outport
  GbADP_3C2Tiout_flg : Outport  Port=2
  GcADP_CabErrInfo_numb : Outport  Port=3
  GcADP_CabCurr_mA : Outport  Port=4
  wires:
  Data Type Conversion1/1 -> ADP_GcADP_CabErrInfo_numb/1
  Data Type Conversion2/1 -> ADP_GbADP_CabErrSt_flg/1
  GcISP_CabErrInfo_numb/1 -> Data Type Conversion1/1  "GcISP_CabErrInfo_numb"
  Relational Operator3/1 -> Logical2/1
  Logical2/1 -> ADP_GbADP_3C2Tiout_flg/1
  Constant10/1 -> Relational Operator3/2
  GbVDP_DiagPermit_flg/1 -> Logical2/2  "GbVDP_DiagPermit_flg"
  GbISP_3C2Tiout_flg/1 -> Relational Operator3/1  "GbISP_3C2Tiout_flg"
  GbISP_CabErrSt_flg/1 -> Data Type Conversion2/1  "GbISP_CabErrSt_flg"
  ADP_GbADP_CabErrSt_flg/1 -> GbADP_CabErrSt_flg/1  "GbADP_CabErrSt_flg"
  ADP_GcADP_CabErrInfo_numb/1 -> GcADP_CabErrInfo_numb/1  "GcADP_CabErrInfo_numb"
  ADP_GbADP_3C2Tiout_flg/1 -> GbADP_3C2Tiout_flg/1  "GbADP_3C2Tiout_flg"
  GcISP_CabCurr_mA/1 -> Sum1/1  "GcISP_CabCurr_mA"
  Sum1/1 -> Data Type Conversion3/1
  ADP_GcADP_CabCurr_mA/1 -> GcADP_CabCurr_mA/1  "GcADP_CabCurr_mA"
  Constant1/1 -> Sum1/2
  Data Type Conversion3/1 -> ADP_GcADP_CabCurr_mA/1

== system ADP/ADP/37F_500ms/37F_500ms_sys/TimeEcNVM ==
  GcADP_YearSet_Yr : Inport
  GcADP_MonthSet_Mn : Inport  Port=2
  GcADP_DaySet_D : Inport  Port=3
  GcADP_HourSet_Hr : Inport  Port=4
  GcADP_MinSet_Min : Inport  Port=5
  GcADP_SecondSet_S : Inport  Port=6
  Enable : EnablePort  StatesWhenEnabling=reset
  Data Store Write : AIWAYS_Powertrain_BMS_lib/Signals/Data Store Write  DSW=EcNVM_ShutdownTimeYr_Yr
  Data Store Write1 : AIWAYS_Powertrain_BMS_lib/Signals/Data Store Write  DSW=EcNVM_ShutdownTimeMonth_M
  Data Store Write2 : AIWAYS_Powertrain_BMS_lib/Signals/Data Store Write  DSW=EcNVM_ShutdownTimeDay_D
  Data Store Write3 : AIWAYS_Powertrain_BMS_lib/Signals/Data Store Write  DSW=EcNVM_ShutdownTimeHr_Hr
  Data Store Write4 : AIWAYS_Powertrain_BMS_lib/Signals/Data Store Write  DSW=EcNVM_ShutdownTimeMint_Min
  Data Store Write5 : AIWAYS_Powertrain_BMS_lib/Signals/Data Store Write  DSW=EcNVM_ShutdownTimeSec_S
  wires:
  GcADP_YearSet_Yr/1 -> Data Store Write/1
  GcADP_MonthSet_Mn/1 -> Data Store Write1/1
  GcADP_DaySet_D/1 -> Data Store Write2/1
  GcADP_HourSet_Hr/1 -> Data Store Write3/1
  GcADP_MinSet_Min/1 -> Data Store Write4/1
  GcADP_SecondSet_S/1 -> Data Store Write5/1

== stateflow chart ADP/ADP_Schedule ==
  (default) -> (junction 50)
  (junction 50) -> (junction 13) : { ADP_050_10ms; ADP_3C2_10ms; ADP_3A0_10ms; }
  (junction 13) -> (junction 150) : { TimeCounter20ms ++; TimeCounter100ms ++; TimeCounter500ms ++; TimeCounter1000ms ++; }
  (junction 150) -> (junction 422) : [TimeCounter20ms >= Const20ms]
  (junction 150) -> (junction 424)
  (junction 422) -> (junction 424) : { ADP_17D_20ms; ADP_195_20ms; ADP_28D_20ms; TimeCounter20ms = 0; }
  (junction 424) -> (junction 503) : [TimeCounter100ms >= Const100ms]
  (junction 424) -> (junction 505)
  (junction 503) -> (junction 505) : {ADP_2AD_100ms; ADP_2BB_100ms; ADP_2DF_100ms; ADP_2F1_100ms; TimeCounter100ms = 0; }
  (junction 505) -> (junction 509) : [TimeCounter500ms >= Const500ms]
  (junction 505) -> (junction 512)
  (junction 509) -> (junction 512) : {ADP_37F_500ms; TimeCounter500ms = 0; }
  (junction 512) -> (junction 533) : [TimeCounter1000ms >= Const1000ms]
  (junction 512) -> (junction 536)
  (junction 533) -> (junction 536) : {ADP_3AA_1000ms; TimeCounter1000ms = 0; }
  data: TimeCounter20ms local uint8; Const100ms constant uint8 =10; TimeCounter100ms local uint8; Const20ms constant uint8 =2; Const500ms constant uint8 =50; TimeCounter500ms local uint8; TimeCounter1000ms local uint8; Const1000ms constant uint8 =100
  events: output FUNCTION_CALL_EVENT; output FUNCTION_CALL_EVENT; output FUNCTION_CALL_EVENT; output FUNCTION_CALL_EVENT; output FUNCTION_CALL_EVENT; output FUNCTION_CALL_EVENT; output FUNCTION_CALL_EVENT; output FUNCTION_CALL_EVENT; output FUNCTION_CALL_EVENT; output FUNCTION_CALL_EVENT; output FUNCTION_CALL_EVENT; output FUNCTION_CALL_EVENT
